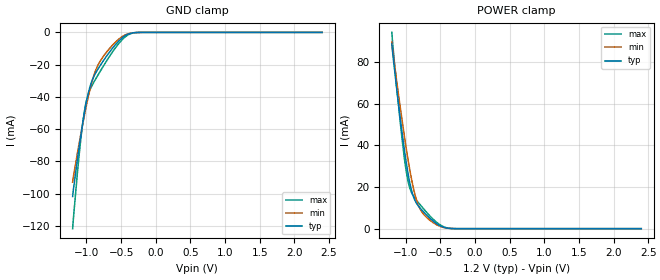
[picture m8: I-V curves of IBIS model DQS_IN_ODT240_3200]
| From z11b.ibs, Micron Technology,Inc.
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| MODEL DQS_IN_ODT240_3200 (Data Strobe Input with 240ohm ODT, 1600-3200Mbps)
[Model]   DQS_IN_ODT240_3200
Model_type   Input
Vinl = 905.000mV
Vinh = 1015.000mV
|   typ   min   max
|C_comp   0.778pF   0.726pF   0.830pF
C_comp_power_clamp   0.389pF   0.363pF   0.415pF
C_comp_gnd_clamp   0.389pF   0.363pF   0.415pF
| Note: C_comp changes when the ODT circuit is enabled.
|[Model Spec]
| Dynamic Overshoot Parameters from DDR4 Specification
|D_overshoot_ampl_h   0.40   NA   NA
|D_overshoot_ampl_l   0.40   NA   NA
|D_overshoot_area_h   0.0800n   NA   NA
|D_overshoot_area_l   0.0800n   NA   NA
[Voltage Range]   1.2000V   1.1400V   1.2600V
| Junction Temperature (Ambient temp is 35C typ, 95C min, 0C max)
[Temperature Range]   50.0   110.0   0.0
[Add Submodel]
| Submodel Name   Mode
240ohm_ODT_3200   Non-Driving
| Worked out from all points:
|   GND clamp passes 1 mA (typ) near -0.39 V on its own axis
|   POWER clamp passes 1 mA (typ) near -0.48 V on its own axis
[GND_clamp]
|   Voltage   I(typ)   I(min)   I(max)
-1.2V     -101.7mA   -92.86mA   -121.7mA
-1.135V   -79.96mA   -75.85mA   -88.92mA
-1.08V    -63.49mA   -62.76mA   -65.41mA
-1.036V   -51.56mA   -52.84mA   -50.64mA
-992.7mV  -41.38mA   -43.58mA   -41.02mA
-927.3mV  -30.76mA   -31.6mA    -33.57mA
-872.7mV  -25.55mA   -24.13mA   -29.29mA
-818.2mV  -21.61mA   -19.01mA   -25.29mA
-621.8mV  -9.659mA   -7.799mA   -11.96mA
-436.4mV  -1.919mA   -1.478mA   -2.611mA
-229.1mV  -17.22uA   -19.75uA   -20.83uA
2.4V      0A         0A         0A
[Power Clamp]
|   Voltage   I(typ)   I(min)   I(max)
-1.2V     88.83mA    89.6mA     94.34mA
-1.135V   68.72mA    72.21mA    70.04mA
-1.058V   47.72mA    53.58mA    44.98mA
-1.004V   34.46mA    41.14mA    30.25mA
-960mV    25.46mA    31.98mA    21.99mA
-894.5mV  16.03mA    20.41mA    16.05mA
-807.3mV  10.5mA     10.53mA    12.15mA
-709.1mV  6.909mA    5.768mA    8.277mA
-545.5mV  2.223mA    1.735mA    2.842mA
-436.4mV  532.9uA    427.3uA    716.1uA
-294.5mV  16.21uA    18.63uA    20.69uA
2.4V      0A         0A         0A
